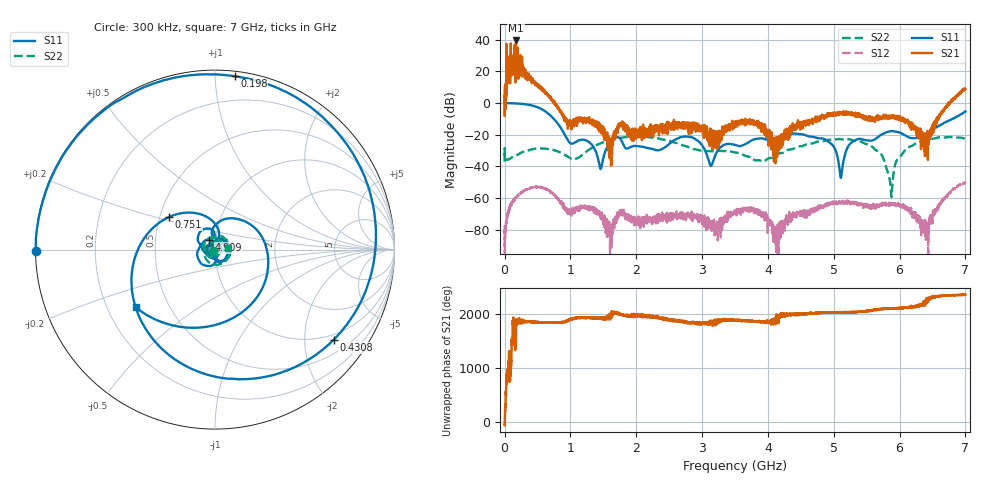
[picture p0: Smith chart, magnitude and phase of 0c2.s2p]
!Keysight Technologies,N5232A,MY52221221,A.10.65.11
!Date: Wednesday, October 16, 2024 12:02:47
!Correction: S11(Full 2 Port(1,4))
!S41(Full 2 Port(1,4))
!S14(Full 2 Port(1,4))
!S44(Full 2 Port(1,4))
!S2P File: Measurements: S11, S41, S14, S44:
# Hz S  RI  R 50
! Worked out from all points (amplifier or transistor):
!   4001 points, 300 kHz to 7 GHz, reference 50 ohm
!   highest |S21| = 39.6 dB at 173.5 MHz (marker M1)
!   |S21| within 3 dB of that: 26.48758 MHz to 26.59825 MHz (110.7 kHz wide, 0.417 % of centre)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
!   unconditionally stable (mu >= 1): 7.334 MHz to 26.19 MHz; 210.5 MHz to 238.3 MHz; 240.2 MHz to end of sweep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
!   at 1.166 GHz: K = 2922.28, MAG = -10.3 dB, |S12| = -65.0 dB
!   at 3.5 GHz: K = 6496.67, MAG = -14.4 dB, |S12| = -67.9 dB
!   at 7 GHz: K = 42.62, MAG = 10.4 dB, |S12| = -50.6 dB
!   S11 on the Smith chart (normalised r, x): 300 kHz: 0.00, -0.00; 198 MHz: 0.03, +1.12; 430.8 MHz: 0.84, -2.73; 751 MHz: 0.56, +0.23; 4.909 GHz: 0.93, +0.10; 7 GHz: 0.32, -0.30
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300000  -0.996 -0.00924  0.8567 -1.482  -0.000121 -6.43e-05  -0.0122 -0.00704
5.62976e7  -0.886 0.4548  7.396 6.484  -0.000219 -0.000266  -0.0139 0.00907
6.32973e7  -0.8573 0.5073  21.76 -7.866  -0.000204 -0.000337  -0.0134 0.0101
1.087954e8  -0.6015 0.7897  -3.558 19.51  -0.000478 -0.000474  -0.01 0.0163
1.297944e8  -0.45 0.8792  -1.242 18.12  -0.000596 -0.000464  -0.00808 0.0186
1.367942e8  -0.3967 0.9042  2.485 12.43  -0.00074 -0.000422  -0.00737 0.0192
1.385441e8  -0.3831 0.9094  15.28 10.81  -0.000682 -0.000366  -0.00728 0.0194
1.490436e8  -0.2992 0.9392  2.446 9.416  -0.00085 -0.000464  -0.00616 0.0203
1.735426e8  -0.0962 0.9751  -4.875 -95.49  -0.00103 -0.000285  -0.00326 0.0221
1.980415e8  0.1094 0.9661  -0.2263 11.11  -0.00117 -0.000143  8.73e-05 0.0236
2.085411e8  0.1962 0.9497  2.027 9.152  -0.00126 -3.03e-05  0.00172 0.024
2.10291e8  0.2104 0.9462  15.37 23.94  -0.0013 -4.72e-05  0.00196 0.0241
2.3479e8  0.405 0.874  8.657 5.275  -0.00136 0.000252  0.00555 0.0254
4.307816e8  0.6606 -0.5029  2.227 3.874  0.000368 0.00214  0.0309 0.0173
7.510178e8  -0.2559 0.1817  0.7635 0.6671  0.000502 -0.00123  0.0241 -0.022
1.1675e9  0.0348 0.0604  -0.1909 0.1837  -0.000358 -0.000307  -0.0179 0.0126
2.3347e9  -0.00354 0.032  -0.1305 0.0436  -0.000164 -0.000177  -0.0406 -0.0651
3.50015e9  -0.0479 0.00217  0.0183 0.1894  -0.000391 -9.97e-05  -0.00776 -0.0265
4.66735e9  -0.0846 0.0177  -0.2098 -0.1727  0.000406 -0.00013  -0.043 -0.0311
4.90884e9  -0.0325 0.0545  -0.27 -0.3453  0.000184 -0.000583  -0.0654 0.0221
5.83455e9  -0.0887 0.09  0.2192 -0.2691  5.77e-05 0.000601  0.00525 -0.000724
7e9  -0.4413 -0.3217  -2.467 -1.285  0.00021 -0.00294  0.0737 0.00982
